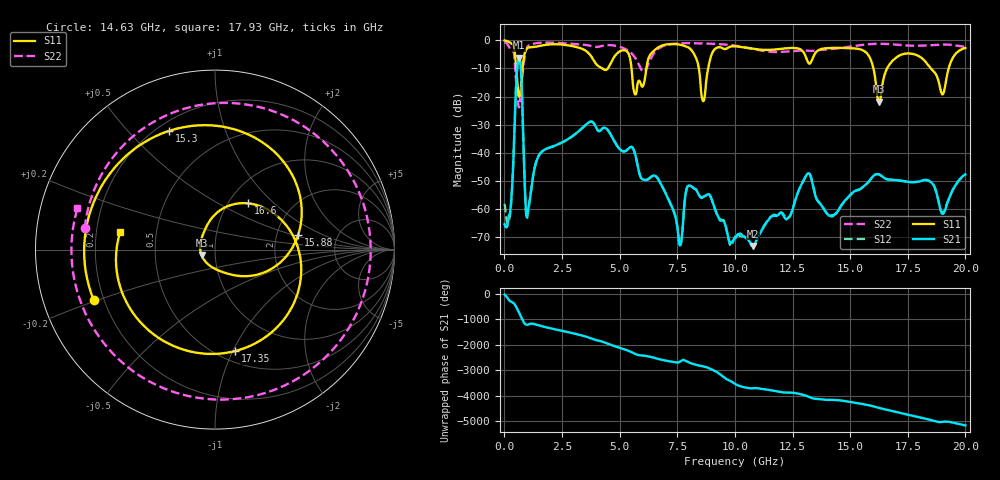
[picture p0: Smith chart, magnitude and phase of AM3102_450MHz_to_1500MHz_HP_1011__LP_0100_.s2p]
!Agilent Technologies,E8364B,MY43040894,A.07.50.67
!Agilent E8364B: A.07.50.67
!Date: Thursday, January 11, 2018 06:23:56
!Correction: S11(Full 2 Port(1,2))
!S21(Full 2 Port(1,2))
!S12(Full 2 Port(1,2))
!S22(Full 2 Port(1,2))
!S2P File: Measurements: S11, S21, S12, S22:
# Hz S  dB  R 50
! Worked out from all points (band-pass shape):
!   1601 points, 10 MHz to 20 GHz, reference 50 ohm
!   highest |S21| = -6.16 dB at 634.7 MHz (marker M1); lowest = -73.1 dB at 10.79 GHz (marker M2)
!   |S21| within 3 dB of the highest: 564.1 MHz to 709.2 MHz (145.1 MHz wide, 22.8 % of centre)
!   lowest |S11| = -21.8 dB at 16.25 GHz (marker M3), VSWR 1.18, Z = 42.9 - j2.64 ohm
!   |S11| at or under -10 dB: 5.516 GHz to 6.16 GHz (643.8 MHz wide, 11 % of centre); 16.01 GHz to 16.6 GHz (591.4 MHz wide, 3.63 % of centre); 18.5 GHz to 19.27 GHz (768.1 MHz wide, 4.07 % of centre)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
!   |S22| runs from -23.8 to -0.5 dB; largest |S21 - S12| = 0.0014
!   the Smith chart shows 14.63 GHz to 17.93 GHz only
!   S11 on the Smith chart (normalised r, x): 14.63 GHz: 0.16, -0.19; 15.3 GHz: 0.25, +0.66; 15.88 GHz: 2.64, +0.54; 16.6 GHz: 1.23, +0.70; 17.35 GHz: 0.60, -1.02; 17.93 GHz: 0.30, +0.08
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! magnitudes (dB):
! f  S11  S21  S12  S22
! 10 MHz  0.0  -65.3  -58.1  -0.5
! 259.9 MHz  -0.9  -60.7  -61.2  -3.3
! 634.7 MHz  -19.9  -6.2  -6.1  -23.8
! 1.01 GHz  -2.7  -61.3  -61.7  -2.2
! 3.346 GHz  -2.9  -31.4  -31.4  -1.5
! 5.682 GHz  -19.3  -40.7  -40.7  -6.3
! 6.682 GHz  -2.5  -49.4  -49.4  -3.0
! 7.619 GHz  -1.6  -72.9  -72.8  -1.1
! 8.618 GHz  -21.6  -55.7  -55.6  -1.1
! 10.01 GHz  -2.1  -70.2  -69.7  -1.9
! 10.79 GHz  -3.0  -73.1  -73.1  -3.1
! 13.34 GHz  -7.1  -49.9  -49.8  -3.8
! 14.63 GHz  -2.7  -58.5  -58.6  -2.7
! 15.3 GHz  -3.0  -53.3  -53.2  -1.9
! 15.88 GHz  -6.6  -49.5  -49.4  -1.4
! 16.25 GHz  -21.8  -47.7  -47.6  -1.2
! 16.6 GHz  -10.0  -49.4  -49.4  -1.3
! 16.68 GHz  -8.9  -49.5  -49.5  -1.3
! 17.35 GHz  -4.8  -50.1  -50.0  -1.8
! 17.93 GHz  -5.4  -50.3  -50.2  -1.9
! 19.01 GHz  -19.2  -61.6  -61.3  -1.5
! 20 GHz  -2.7  -47.6  -47.8  -2.3
